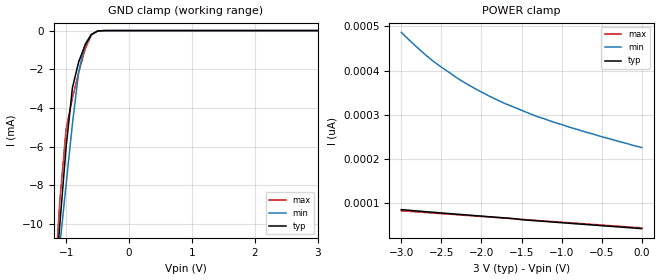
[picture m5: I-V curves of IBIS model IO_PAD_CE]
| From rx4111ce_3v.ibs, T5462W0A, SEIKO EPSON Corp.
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[Model]   IO_PAD_CE
Model_type Input
Enable Active-High
Polarity Non-Inverting
Vinh=2.64
Vinl=0.54
C_comp   2.5p   2.0p   3.0p
[Temperature Range] 25   105   -40
[Voltage Range]   3.0   2.7   3.3
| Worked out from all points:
|   GND clamp passes 1 mA (typ) near -0.73 V on its own axis
[GND Clamp]
-3V       -88.87mA   -72.8mA    -108mA
-1.2V     -14.09mA   -14.29mA   -13.9mA
-1.1V     -10.01mA   -11.11mA   -8.777mA
-1V       -6.002mA   -7.943mA   -5.058mA
-900mV    -2.958mA   -4.822mA   -3.504mA
-800mV    -1.61mA    -2.135mA   -2.158mA
-700mV    -762.7uA   -702uA     -983.6uA
-600mV    -207.8uA   -197.3uA   -229uA
-500mV    -21.89uA   -34.52uA   -13.51uA
-300mV    -47.04nA   -340.8nA   -3.548nA
3V        42.19pA    240.2pA    40.04pA
[POWER Clamp]
-3V       85.32pA    486.4pA    82.47pA
-2.7V     80.67pA    435.8pA    78.73pA
-2.6V     79.22pA    420.8pA    77.45pA
-2.5V     77.77pA    407.7pA    76.14pA
-2.3V     74.86pA    382.6pA    73.55pA
-2.2V     73.43pA    371.6pA    72.33pA
-2V       70.62pA    351.4pA    69.63pA
-1.8V     67.79pA    333.2pA    67.17pA
-1.4V     61.13pA    302.7pA    62.08pA
-1.1V     56.98pA    283.2pA    58.19pA
-500mV    48.89pA    250.3pA    50.38pA
0V        42.19pA    225.8pA    43.94pA
